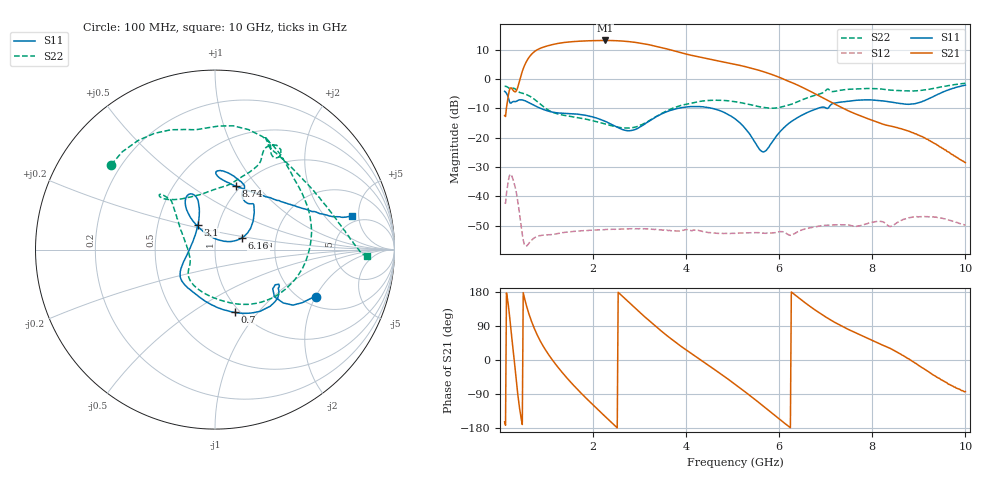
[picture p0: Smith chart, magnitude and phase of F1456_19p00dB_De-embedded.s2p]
! Integrated Device Technology
! Corporate Headquarters
! 6024 Silver Creek Valley Road
! San Jose, CA 95138  USA
! Phone:  1-408-284-8200
! Toll Free:  1-800-223-1366
! Webpage:  http://www.idt.com/
! Timing and RF Division
! 515 Groton Road, Suite 102
! Westford, MA 01886-6024
! Device:  F1456
! Description: 6-bit 0.5 dB Transmit Variable Gain Amplifier
! Frequency:  2100.0 -  2950.00 MHz
! Package:  6x6 mm Thin QFN Plastic Package: 28 pin
! State:  38
! Atten State:  19.0 dB
! Voltage:  +5.00 Volts
! Current:  216.982 mA
! Data:  The device was measured on a the F1455 evaluation board which has
!  individual transmission lines to the RF pins.  Data was collected
!  using a calibrated network analyzer.  The evaluation board was
!  de-embedded using a TRL calibration technique.
!  The reference plane is the edge of the package pin.
!  Pin  1 = CSb
!  Pin  2 = DATA
!  Pin  3 = CLK
!  Pin  4 = RSET
!  Pin  5 = GND
!  Pin  6 = RFIN  = Port 1
!  Pin  7 = GND
!  Pin  8 = NC
!  Pin  9 = NC
!  Pin 10 = NC
!  Pin 11 = NC
!  Pin 12 = NC
!  Pin 13 = NC
!  Pin 14 = /STBY
!  Pin 15 = GND
!  Pin 16 = RFOUT  = Port 2
!  Pin 17 = GND
!  Pin 18 = NC
!  Pin 19 = NC
!  Pin 20 = NC
!  Pin 21 = GND
!  Pin 22 = NC
!  Pin 23 = GND
!  Pin 24 = NC
!  Pin 25 = NC
!  Pin 26 = NC
!  Pin 27 = GND
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# GHz S dB R 50
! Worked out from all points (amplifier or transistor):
!   496 points, 100 MHz to 10 GHz, reference 50 ohm
!   highest |S21| = 13.1 dB at 2.26 GHz (marker M1)
!   |S21| within 3 dB of that: 820.7 MHz to 3.615 GHz (2.794 GHz wide, 126 % of centre)
!   unconditionally stable (mu >= 1): start of sweep to end of sweep
!   at 1.74 GHz: K = 39.04, MAG = 13.4 dB, |S12| = -51.7 dB
!   at 5.06 GHz: K = 95.38, MAG = 5.9 dB, |S12| = -52.5 dB
!   at 10 GHz: K = 449.03, MAG = -18.9 dB, |S12| = -49.8 dB
!   S11 on the Smith chart (normalised r, x): 100 MHz: 2.36, -2.00; 700 MHz: 0.95, -0.76; 3.1 GHz: 0.80, +0.23; 6.16 GHz: 1.34, +0.18; 8.74 GHz: 0.95, +0.78; 10 GHz: 4.18, +4.09
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0.1  -4.18 -25.0  -12.45 -163.6  -42.30 49.0  -2.53 140.8
0.3  -7.66 -30.8  -4.18 7.8  -35.22 -133.9  -3.17 74.5
0.42  -7.10 -37.7  -0.61 -126.2  -45.82 140.8  -4.57 41.6
0.56  -7.59 -56.5  5.68 147.5  -56.94 151.3  -5.23 10.6
0.7  -8.72 -72.6  8.77 95.0  -54.58 143.1  -6.46 -20.7
0.94  -10.43 -96.6  10.89 34.2  -53.18 98.8  -9.51 -65.4
1.16  -11.37 -113.9  11.84 -5.4  -52.90 73.9  -11.49 -92.6
1.48  -11.76 -131.3  12.61 -53.1  -52.09 48.5  -12.66 -119.4
1.76  -12.17 -141.8  12.92 -89.5  -51.68 31.4  -13.41 -133.0
2  -12.96 -148.6  13.06 -118.5  -51.49 18.7  -14.23 -140.1
2.26  -14.43 -158.1  13.12 -149.0  -51.27 6.2  -15.33 -146.5
2.64  -17.27 174.2  12.91 167.0  -51.12 -11.2  -16.65 -161.6
3.1  -15.46 124.0  11.97 115.1  -51.01 -33.1  -15.15 163.6
3.4  -12.51 111.6  10.97 83.2  -51.30 -46.9  -12.42 145.8
4.08  -9.41 113.3  8.18 19.8  -51.57 -77.5  -8.33 132.1
5.06  -13.67 127.7  4.95 -64.8  -52.54 -123.8  -7.74 135.6
5.66  -24.86 70.7  2.50 -121.9  -52.49 -160.2  -9.69 118.0
6.16  -15.72 23.9  -0.51 -171.2  -52.70 166.4  -9.05 82.8
6.7  -10.77 41.5  -4.46 138.1  -50.55 144.0  -5.90 63.9
8.36  -7.75 88.1  -15.94 32.2  -50.14 69.9  -3.76 62.5
8.74  -8.57 72.1  -17.58 5.5  -47.47 65.6  -4.07 49.2
10  -2.10 13.9  -28.48 -83.3  -49.78 -22.9  -1.46 -2.6
